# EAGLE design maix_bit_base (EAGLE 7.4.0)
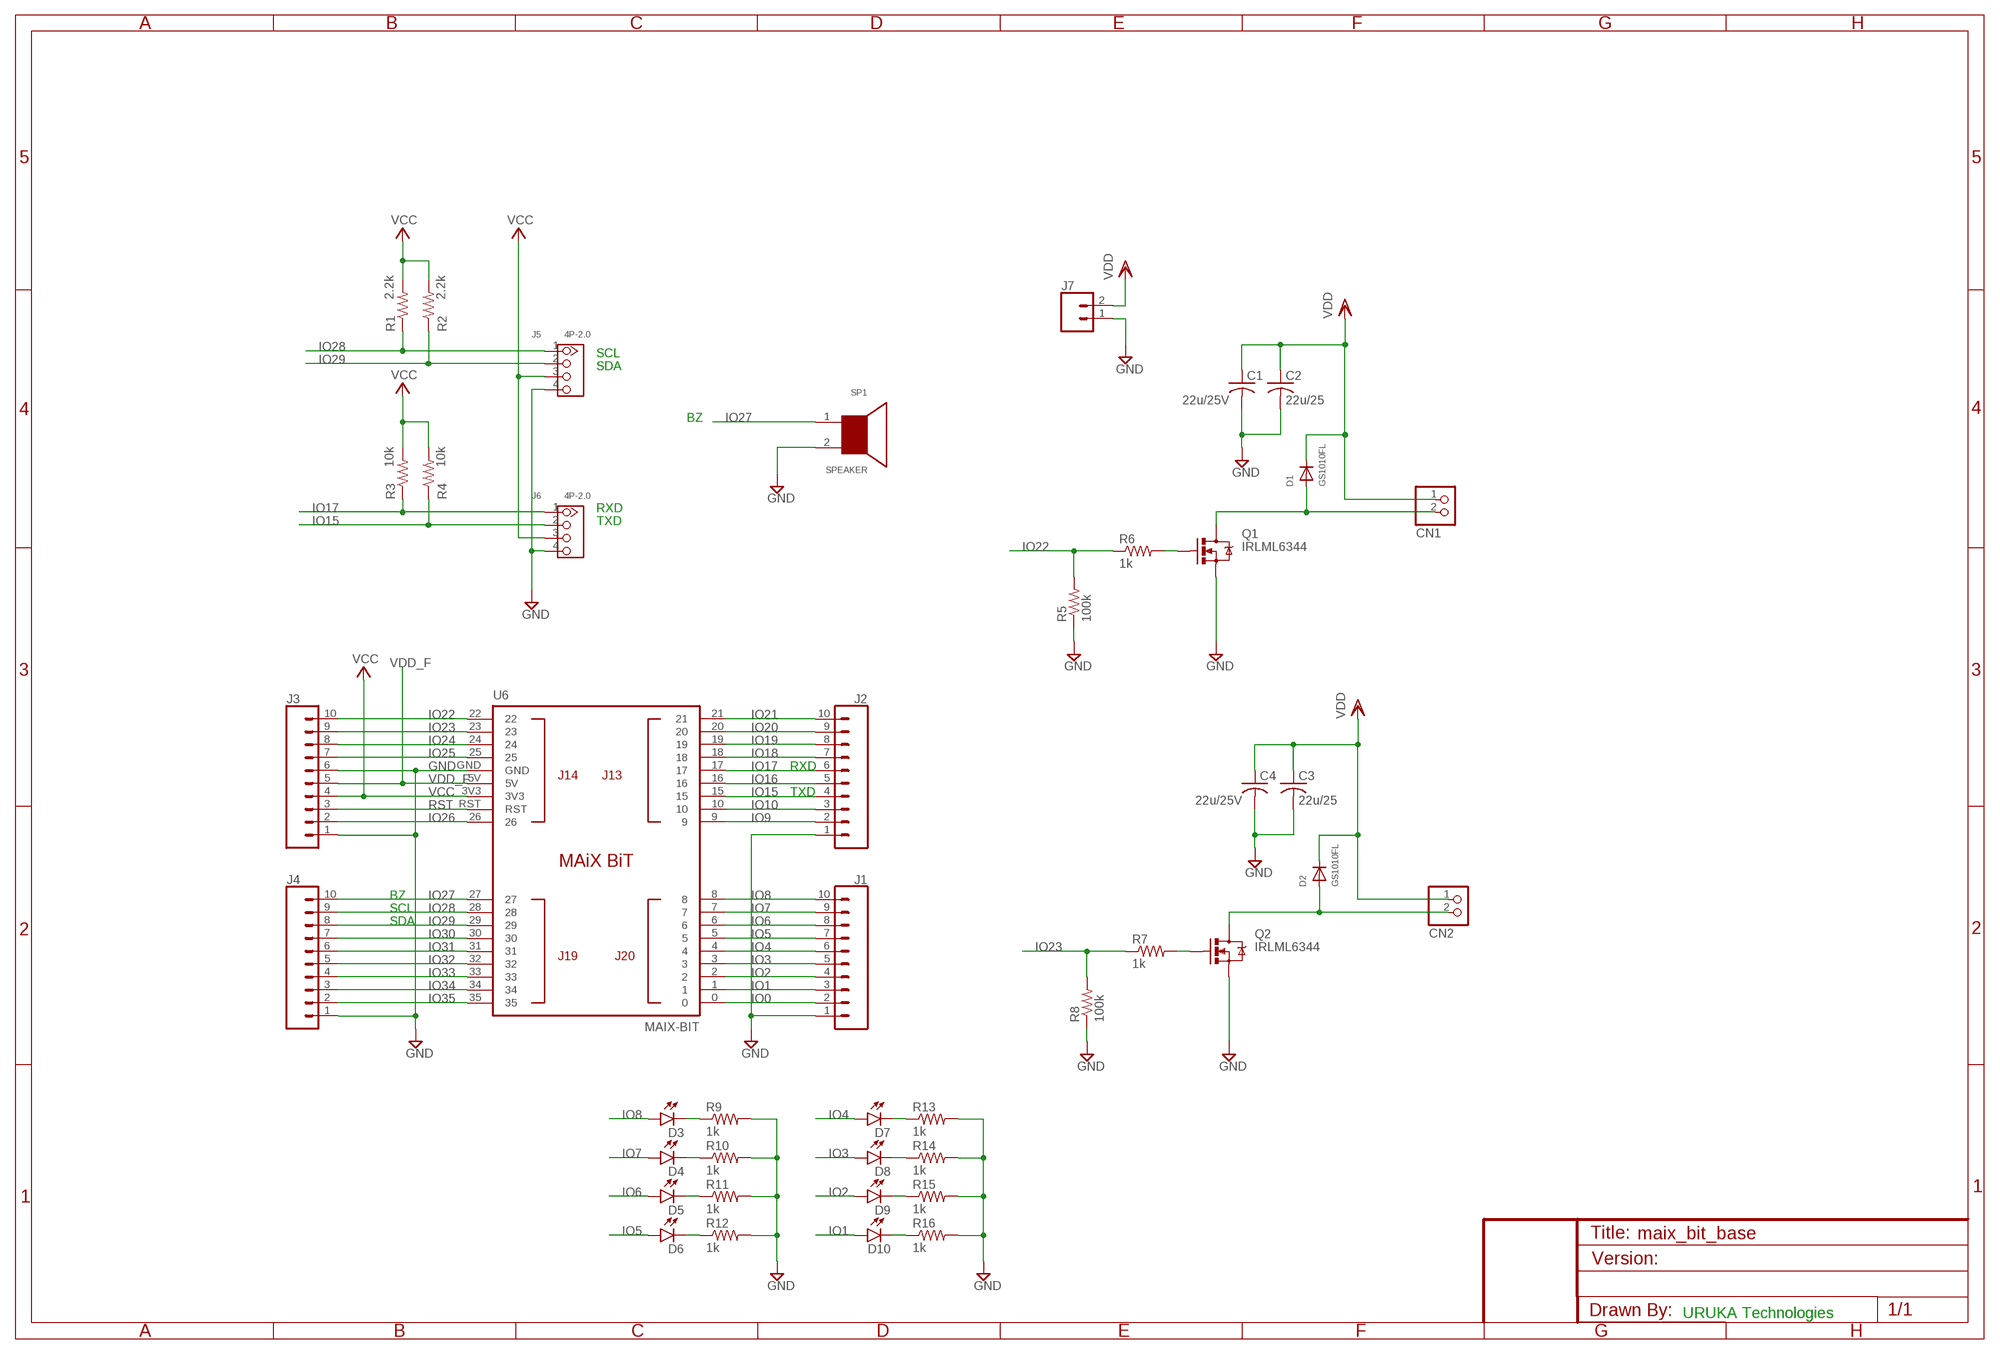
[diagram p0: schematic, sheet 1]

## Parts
C1  22u/25V  C-USC0805  [C0805]
C2  22u/25  C-USC0805  [C0805]
C3  22u/25  C-USC0805  [C0805]
C4  22u/25V  C-USC0805  [C0805]
CN1  JST_2PIN-SMT-RA  [JST-PH-2-SMT-RA]
CN2  JST_2PIN-SMT-RA  [JST-PH-2-SMT-RA]
D1  GS1010FL  [SOD-123FL]
D2  GS1010FL  [SOD-123FL]
D3  LED0603  [LED-0603]
D4  LED0603  [LED-0603]
D5  LED0603  [LED-0603]
D6  LED0603  [LED-0603]
D7  LED0603  [LED-0603]
D8  LED0603  [LED-0603]
D9  LED0603  [LED-0603]
D10  LED0603  [LED-0603]
J1  CONN_10"  [1X10]
J2  CONN_10"  [1X10]
J3  CONN_10"  [1X10]
J4  CONN_10"  [1X10]
J5  4P-2.0  GROVE-CONNECTOR-DIP(4P-2.0)  [HW4-2.0]
J6  4P-2.0  GROVE-CONNECTOR-DIP(4P-2.0)  [HW4-2.0]
J7  CONN_02  [1X02]
Q1  IRLML6344  MOSFET-NCHANNELBSS138  [SOT23-3]
Q2  IRLML6344  MOSFET-NCHANNELBSS138  [SOT23-3]
R1  2.2k  R-US_R0603  [R0603]
R2  2.2k  R-US_R0603  [R0603]
R3  10k  R-US_R0603  [R0603]
R4  10k  R-US_R0603  [R0603]
R5  100k  R-US_R0603  [R0603]
R6  1k  R-US_R0603  [R0603]
R7  1k  R-US_R0603  [R0603]
R8  100k  R-US_R0603  [R0603]
R9  1k  R-US_R0603  [R0603]
R10  1k  R-US_R0603  [R0603]
R11  1k  R-US_R0603  [R0603]
R12  1k  R-US_R0603  [R0603]
R13  1k  R-US_R0603  [R0603]
R14  1k  R-US_R0603  [R0603]
R15  1k  R-US_R0603  [R0603]
R16  1k  R-US_R0603  [R0603]
SP1  SPEAKER  [SPEAKER]
U6  MAIX-BIT  [MAIX-BIT]

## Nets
GND [power]: C1.2 C2.2 C3.2 C4.2 J1.1 J2.1 J3.1 J3.6 J4.1 J5.4 J6.4 J7.1 Q1.2(S) Q2.2(S) R5.1 R8.1 R9.2 R10.2 R11.2 R12.2 R13.2 R14.2 R15.2 R16.2 SP1.2 U6.GND
IO0: J1.2 U6.0
IO1: D10.A J1.3 U6.1
IO2: D9.A J1.4 U6.2
IO3: D8.A J1.5 U6.3
IO4: D7.A J1.6 U6.4
IO5: D6.A J1.7 U6.5
IO6: D5.A J1.8 U6.6
IO7: D4.A J1.9 U6.7
IO8: D3.A J1.10 U6.8
IO9: J2.2 U6.9
IO10: J2.3 U6.10
IO15: J2.4 J6.2 R4.1 U6.15
IO16: J2.5 U6.16
IO17: J2.6 J6.1 R3.1 U6.17
IO18: J2.7 U6.18
IO19: J2.8 U6.19
IO20: J2.9 U6.20
IO21: J2.10 U6.21
IO22: J3.10 R5.2 R6.1 U6.22
IO23: J3.9 R7.1 R8.2 U6.23
IO24: J3.8 U6.24
IO25: J3.7 U6.25
IO26: J3.2 U6.26
IO27: J4.10 SP1.1 U6.27
IO28: J4.9 J5.1 R1.1 U6.28
IO29: J4.8 J5.2 R2.1 U6.29
IO30: J4.7 U6.30
IO31: J4.6 U6.31
IO32: J4.5 U6.32
IO33: J4.4 U6.33
IO34: J4.3 U6.34
IO35: J4.2 U6.35
N$9: Q2.1(G) R7.2
N$10: Q1.1(G) R6.2
N$11 [moter]: CN1.2 D1.A Q1.3(D)
N$12 [moter]: CN2.2 D2.A Q2.3(D)
N$13: D4.C R10.1
N$14: D5.C R11.1
N$15: D6.C R12.1
N$16: D7.C R13.1
N$17: D8.C R14.1
N$18: D9.C R15.1
N$19: D10.C R16.1
N$20: D3.C R9.1
RST: J3.3 U6.RST
VCC [power]: J3.4 J5.3 J6.3 R1.2 R2.2 R3.2 R4.2 U6.3V3
VDD [moter]: C1.1 C2.1 C3.1 C4.1 CN1.1 CN2.1 D1.C D2.C J7.2
VDD_F [power]: J3.5 U6.5V

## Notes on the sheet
- SCL
- SDA
- BZ
- RXD
- TXD
- RXD
- TXD
- BZ
- SCL
- SDA
- URUKA Technologies

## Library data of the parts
C1-C4 = adafruit:C-US: CAPACITOR, American symbol
CN1 CN2 = solecon:JST_2PIN: JST 2-Pin Connectors of various flavors
D1 D2 = suna_power_device:GS1010FL
D3-D10 = SparkFun-LED:LED: LEDs
J1-J4 = SparkFun-Connectors:CONN_10: Multi connection point. Often used as Generic Header-pin footprint for 0.1 inch spaced/style header connections On any of the 0.1 inch spaced packages, you can populate with these: Break Away Headers - Straight (PRT-00116) Break Away Male Headers - Right Angle (PRT-00553) Female Headers (PRT-00115)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; PROD_ID: CONN-11563
J5 J6 = Seeed-OPL-Connector:GROVE-CONNECTOR-DIP(4P-2.0): 320110033
J7 = SparkFun-Connectors:CONN_02: Multi connection point. Often used as Generic Header-pin footprint for 0.1 inch spaced/style header connections
Q1 Q2 = SparkFun-DiscreteSemi:MOSFET-NCHANNEL: Common NMOSFET Parts MFG P/NStore IDProd ID FDD8780TRANS-09984 SI7820DNTRANS-11055 FDS6630AIC-08089 2N7002PWTRANS-11151 FQP30N06L COM-10213TRANS-10060 BSS123LT1GTRANS-08345 BSS138TRANS-00830 BS170 2N7000; PROD_ID: TRANS-00830; VALUE: 200mA/50V
R1-R16 = resistor:R-US_: RESISTOR, American symbol
SP1 = cq:SPEAKER
U6 = solecon:MAIX-BIT

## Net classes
1 power: width 0.762 mm, clearance 0.254 mm
2 Neopix: width 0.356 mm
3 moter: width 0.762 mm, clearance 0.254 mm

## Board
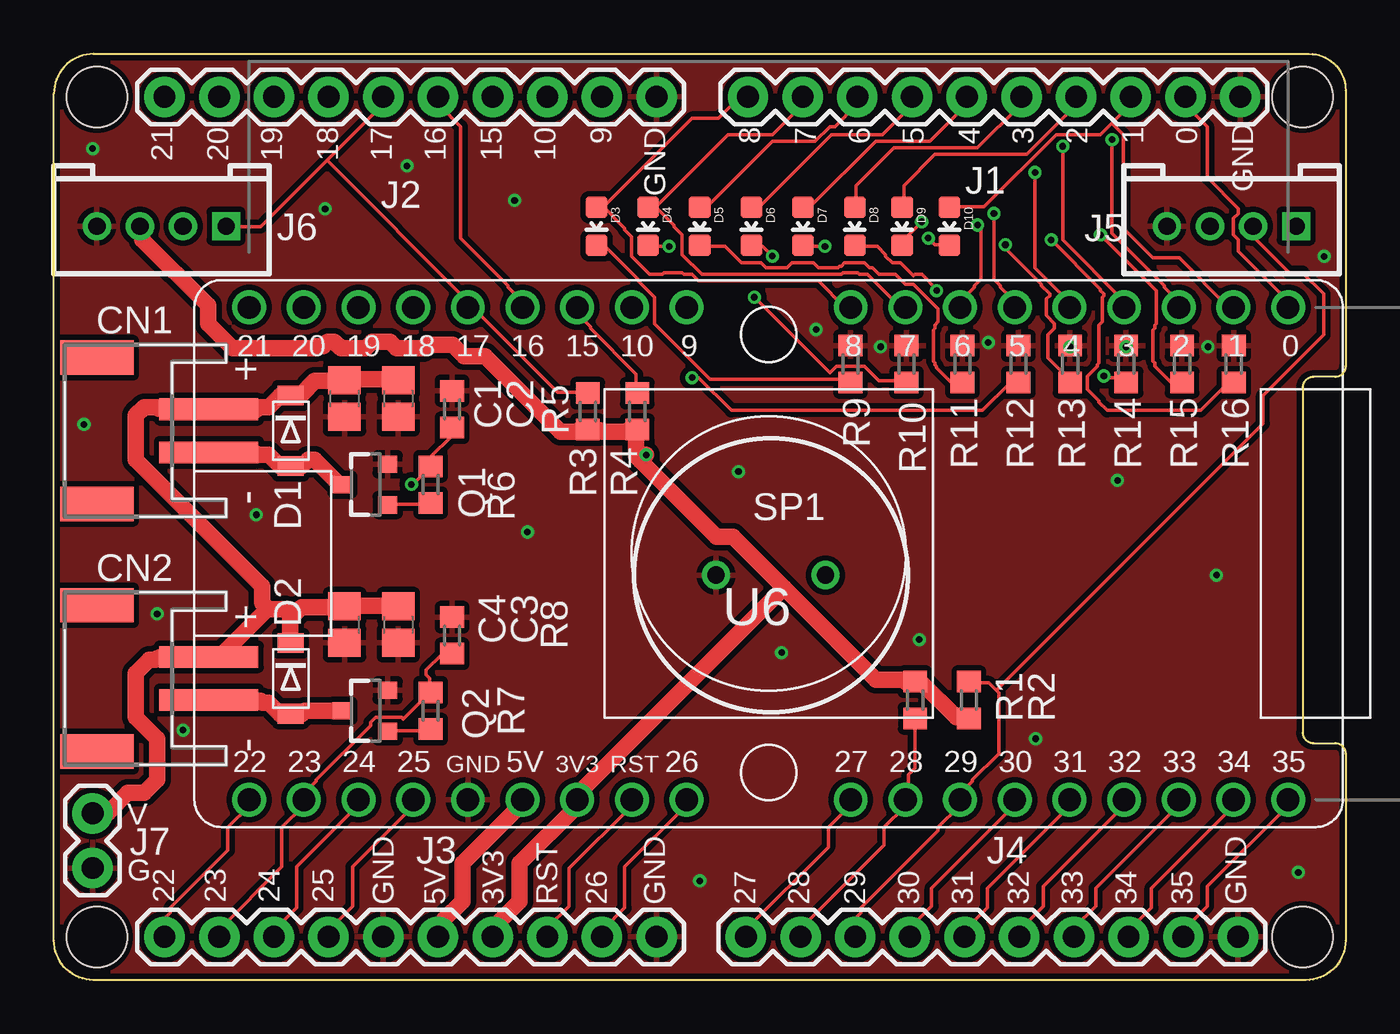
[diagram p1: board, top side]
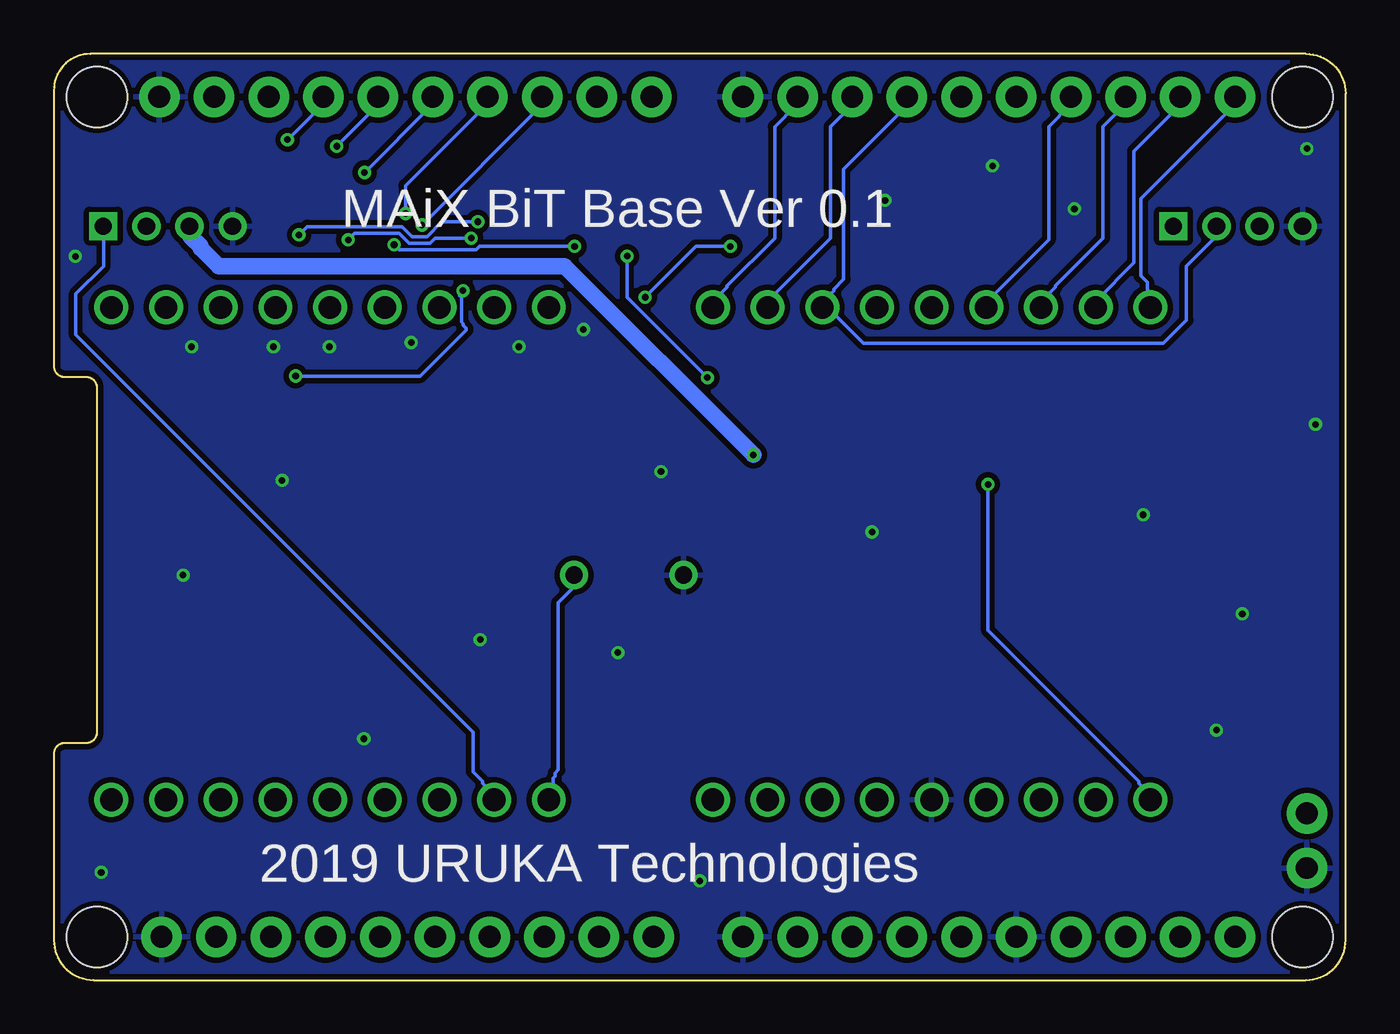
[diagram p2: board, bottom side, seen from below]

Size 60 x 43 mm. Coordinates in mm from the lower left corner, seen from the top.
Outline: 1.84,43 58.3,43 arc-90 60,41.3 60,28.5 arc-90 59.5,28 58.5,28 arc90 58,27.5 58,11.5 arc90 58.5,11 59.5,11 arc-90 60,10.5 60,1.84 arc-90 58.16,0 1.84,0 arc-90 0,1.84 0,41.16 arc-90 1.84,43
Copper layers (1*16): Top 0.035mm / dielectric 1.5mm / Bottom 0.035mm
Design rules "ssci_SeeedStudio_2layer_DRU_no_angle": minimum track width 6mil, minimum drill 12mil, track to track 6mil, track to pad 6mil, pad to pad 6mil, via to via 6mil, smd to smd 0mil, copper to edge 10mil, drill to drill 10mil, minimum pad ring 10mil, minimum via ring 6mil, stop-mask expansion 2mil, vias tented up to drill 25mil, thermal gap 10mil
Holes 2.8 mm at 2,41 2,2 58,2 58,41

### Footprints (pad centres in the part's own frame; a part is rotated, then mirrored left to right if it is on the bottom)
C0805 = smd 1.3 x 1.5: 1 -0.85,0; 2 0.85,0
JST-PH-2-SMT-RA = smd 1 x 4.6: 1 1,-3.7; 2 -1,-3.7 | smd 1.6 x 3.4: NC1 -3.4,1.5; NC2 3.4,1.5
SOD-123FL = smd 0.91 x 1.22: A 1.637,0; C -1.637,0
LED-0603 = smd 1 x 1: A 0,-0.877; C 0,0.877
1X10 = drill 1.016 pad 1.88: 1 0,0; 2 2.54,0; 3 5.08,0; 4 7.62,0; 5 10.16,0; 6 12.7,0; 7 15.24,0; 8 17.78,0; 9 20.32,0; 10 22.86,0
HW4-2.0 = drill 0.8 pad 1.27 square: 1 -3,0 | drill 0.8 pad 1.27: 2 -1,0; 3 1,0; 4 3,0
1X02 = drill 1.016 pad 1.88: 1 0,0; 2 2.54,0
SOT23-3 = smd 0.8 x 0.9: 1 -0.95,-1; 2 0.95,-1; 3 0,1.1
R0603 = smd 1 x 1.1: 1 -0.85,0; 2 0.85,0
SPEAKER = drill 0.8: 1 -2.54,0; 2 2.54,0
MAIX-BIT = drill 1.05: 0 24.13,11.43; 1 21.59,11.43; 2 19.05,11.43; 3 16.51,11.43; 3V3 -8.89,-11.43; 4 13.97,11.43; 5 11.43,11.43; 5V -11.43,-11.43; 6 8.89,11.43; 7 6.35,11.43; 8 3.81,11.43; 9 -3.81,11.43; 10 -6.35,11.43; 15 -8.89,11.43; 16 -11.43,11.43; 17 -13.97,11.43; 18 -16.51,11.43; 19 -19.05,11.43; 20 -21.59,11.43; 21 -24.13,11.43; 22 -24.13,-11.43; 23 -21.59,-11.43; 24 -19.05,-11.43; 25 -16.51,-11.43; 26 -3.81,-11.43; 27 3.81,-11.43; 28 6.35,-11.43; 29 8.89,-11.43; 30 11.43,-11.43; 31 13.97,-11.43; 32 16.51,-11.43; 33 19.05,-11.43; 34 21.59,-11.43; 35 24.13,-11.43; GND -13.97,-11.43; RST -6.35,-11.43

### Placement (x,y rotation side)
C1  13.5,27 270 top
C2  16,27 270 top
C3  16,16.5 270 top
C4  13.5,16.5 270 top
CN1  3.5,25.5 90 top
CN2  3.5,14 90 top
D1  11,25.5 270 top
D2  11,14 270 top
D3  25.2,35 180 top
D4  27.6,35 180 top
D5  30,35 180 top
D6  32.4,35 180 top
D7  34.8,35 180 top
D8  37.2,35 180 top
D9  39.4,35 180 top
D10  41.6,35 180 top
J1  55.1,41 180 top
J2  28,41 180 top
J3  28,2 180 top
J4  55,2 180 top
J5  54.7,35 180 top
J6  5,35 180 top
J7  1.8,5.2 90 top
Q1  14.5,23 90 top
Q2  14.5,12.5 90 top
R1  40,13 90 top
R2  42.5,13 270 top
R3  24.8,26.4 270 top
R4  27.1,26.4 270 top
R5  18.5,26.5 270 top
R6  17.5,23 270 top
R7  17.5,12.5 270 top
R8  18.5,16 270 top
R9  37,28.6 90 top
R10  39.6,28.6 90 top
R11  42.2,28.6 90 top
R12  44.8,28.6 90 top
R13  47.2,28.6 90 top
R14  49.8,28.6 90 top
R15  52.4,28.6 90 top
R16  54.8,28.6 90 top
SP1  33.3,18.8 180 top
U6  33.2,19.8 0 top

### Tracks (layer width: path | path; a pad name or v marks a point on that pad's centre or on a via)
GND  (via drill 0.3)
  other vias: 1.8,38.6 16.4,37.8 21.4,36.2 12.6,35.8 1.4,25.8 9.4,21.6 22,20.8 31.8,23.6 49.4,23.2 54,18.8 40.2,15.8 33.8,15.2 30,4.6 57.8,5 6,11.6 4.8,17 59,33.6 45.6,11.2 43.4,29.6 53.6,29.4 38.4,29.4 35.4,30.2 49.8,29.4 47.2,29.4
  pour Top: 0,0 60,0 60,43 0,43
  pour Bottom: 0,0 60,0 60,43 0,43
IO0
  Top 0.152: U6.0 57.3,31.24 57.3,31.55 55.02,33.83 55.02,34.37 54.79,34.59 54.79,35.36 55.02,35.59 55.02,35.81 53.57,37.26 53.57,39.62 52.58,40.62 52.58,41 J1.2
IO1
  Top 0.152: 49.15,39.78 49.99,40.62 49.99,41 J1.3 | 49.15,39.78 48.62,39.24 46.56,39.24 43.2,35.89 D10.A | 49.15,39.78 49.68,39.24 49.68,34.9 51.05,33.53 52.27,33.53 54.56,31.24 54.79,31.24 U6.1
IO2  (via drill 0.3)
  Top 0.152: D9.A 39.47,35.89 39.47,36.88 40.92,38.33 45.19,38.33 47.47,40.62 J1.4 | v49.15,39.01 49.15,34.67 51.59,32.23 51.59,32.16 52.2,31.55 52.2,31.24 U6.2
  Bottom 0.152: v49.15,39.01 47.55,40.62 47.55,41 J1.4
IO3  (via drill 0.3)
  Top 0.152: D8.A 37.26,35.89 37.26,36.88 39.01,38.63 42.9,38.63 44.88,40.62 44.88,41 J1.5 | v46.86,38.71 46.86,34.37 49.68,31.55 49.68,31.24 U6.3
  Bottom 0.152: v46.86,38.71 44.96,40.62 44.96,41 J1.5
IO4  (via drill 0.3)
  Top 0.152: D7.A 34.82,35.89 35.13,35.89 38.18,38.94 40.69,38.94 42.37,40.62 42.37,41 J1.6 | v45.57,37.49 45.57,33.07 47.17,31.47 47.17,31.24 U6.4
  Bottom 0.152: v45.57,37.49 42.44,40.62 42.44,41 J1.6
IO5  (via drill 0.3)
  Top 0.152: D6.A 32.46,35.89 32.77,35.89 36.12,39.24 38.48,39.24 39.85,40.62 J1.7 | v43.66,35.59 43.66,32.54 43.97,32.23 43.97,32.16 44.58,31.55 44.58,31.24 U6.5
  Bottom 0.152: v43.66,35.59 43.66,36.88 39.93,40.62 39.93,41 J1.7
IO6  (via drill 0.3)
  Top 0.152: D5.A 30.02,35.89 30.33,35.89 33.38,38.94 35.36,38.94 36.04,39.62 36.27,39.62 37.26,40.62 37.26,41 J1.8 | v42.9,35.05 43.05,34.9 43.05,32.54 42.75,32.23 42.75,32.16 42.14,31.55 42.14,31.24 U6.6
  Bottom 0.152: v42.9,35.05 37.34,40.62 37.34,41 J1.8
IO7
  Top 0.152: 27.89,35.89 27.96,35.89 31.32,39.24 33.38,39.24 34.75,40.62 34.75,41 J1.9 | 27.89,35.89 27.66,35.89 D4.A 27.89,35.89 | 27.89,35.89 27.96,35.81 28.04,35.81 28.8,35.05 28.8,34.98 29.18,34.59 29.18,33.68 30.1,32.77 36.58,32.77 36.65,32.84 37.34,32.84 37.41,32.77 37.8,32.77 39.32,31.24 39.55,31.24 U6.7
IO8
  Top 0.152: 25.53,35.89 25.22,35.89 D3.A 25.53,35.89 | 25.53,35.89 29.64,40.01 30.86,40.01 31.85,41 J1.10 | 25.53,35.89 26.52,34.9 26.52,34.82 26.82,34.52 26.82,33.6 27.66,32.77 28.27,32.77 28.35,32.84 29.18,32.84 29.26,32.77 29.64,32.77 29.95,32.46 35.51,32.46 36.73,31.24 36.96,31.24 U6.8
IO9
  Bottom 0.152: U6.9 29.34,31.24 29.34,31.55 28.73,32.16 28.73,32.23 26.52,34.44 26.52,39.62 25.53,40.62 25.53,41 J2.2
IO10
  Bottom 0.152: U6.10 26.82,31.24 26.82,31.55 23.93,34.44 23.93,39.62 22.94,40.62 22.94,41 J2.3
IO15
  Top 0.152: R4.1 27.05,27.28 27.05,28.12 24.92,30.25 24.92,30.33 24.38,30.86 24.38,31.17 U6.15
  Bottom 0.152: J6.2 6.02,34.98 6.02,34.52 7.39,33.15 7.39,30.63 8.46,29.57 22.4,29.57 24,31.17 24.31,31.17 U6.15 23.93,31.17 23.93,31.85 23.77,32 23.77,32.08 23.32,32.54 23.32,37.64 20.42,40.54 20.42,41 J2.4
IO16
  Top 0.152: U6.16 21.72,31.24 21.72,31.55 21.11,32.16 21.11,32.23 18.9,34.44 18.9,39.62 17.91,40.62 17.91,41 J2.5
IO17
  Top 0.152: R3.1 24.77,27.28 23.39,27.28 19.51,31.17 19.28,31.17 U6.17 19.2,31.24 19.2,31.55 12.69,38.06 | 12.69,38.06 15.24,40.62 15.24,41 J2.6 | 12.69,38.06 9.6,34.98 8,34.98 J6.1
IO18
  Bottom 0.152: U6.18 16.69,31.24 16.69,31.47 13.79,34.37 13.79,39.62 12.8,40.62 12.8,41 J2.7
IO19
  Bottom 0.152: U6.19 14.1,31.24 14.1,31.55 13.49,32.16 13.49,32.23 11.28,34.44 11.28,39.62 10.29,40.62 10.29,41 J2.8
IO20
  Bottom 0.152: U6.20 11.58,31.24 11.58,31.55 9.83,33.3 9.83,38.48 7.7,40.62 7.7,41 J2.9
IO21
  Bottom 0.152: U6.21 9.14,31.24 9.14,32 9.22,32.08 9.22,32.38 9.53,32.69 9.53,36.27 5.18,40.62 5.18,41 J2.10
IO22  (via drill 0.3)
  Top 0.152: R5.2 18.44,25.6 18.44,25.22 17.53,24.31 17.53,23.85 R6.1 17.45,23.77 16.69,23.01 v16.61,23.01 | J3.10 5.18,2.06 5.18,2.9 5.41,3.12 5.41,3.35 8.08,6.02 8.08,7.09 9.07,8.08 9.07,8.31 U6.22
  Bottom 0.152: v16.61,23.01 16.61,16.23 9.6,9.22 9.6,9.14 9.14,8.69 9.14,8.38 U6.22
IO23
  Top 0.152: R8.2 18.44,15.09 17.98,15.09 17.3,14.4 17.3,14.17 17.45,14.02 17.45,13.41 R7.1 17.45,13.34 16.23,12.12 16.15,12.19 14.94,12.19 14.71,11.96 14.71,11.81 12.19,9.3 12.19,9.22 11.66,8.69 11.66,8.38 U6.23 11.58,8.31 11.58,8.08 10.59,7.09 10.59,5.26 7.7,2.36 7.7,2.06 J3.9
IO24
  Top 0.152: U6.24 14.1,8.31 14.1,8.08 11.28,5.26 11.28,3.35 10.29,2.36 10.29,2.06 J3.8
IO25
  Top 0.152: U6.25 16.69,8.31 16.69,8.08 13.87,5.26 13.87,3.43 12.8,2.36 12.8,2.06 J3.7
IO26
  Top 0.152: U6.26 29.34,8.31 29.34,8.08 26.52,5.26 26.52,3.35 25.53,2.36 25.53,2.06 J3.2
IO27
  Top 0.152: J4.10 32.16,2.06 32.16,2.36 35.97,6.17 35.97,7.09 36.96,8.08 36.96,8.31 U6.27
  Bottom 0.152: SP1.1 35.89,18.75 35.89,18.21 36.58,17.53 36.58,9.75 36.73,9.6 36.73,9.45 36.8,9.37 36.8,9.14 36.96,8.99 36.96,8.38 U6.27
IO28
  Top 0.152: R1.1 40.01,12.12 40.01,9.83 39.7,9.53 39.7,8.46 39.62,8.38 U6.28 39.55,8.31 39.55,8.08 38.56,7.09 38.56,6.25 34.75,2.44 34.75,2.06 J4.9
  Bottom 0.152: J5.1 57.68,34.98 57.68,33.15 58.98,31.85 58.98,29.95 40.54,11.51 40.54,9.68 40.08,9.22 40.08,9.14 39.62,8.69 39.62,8.38 U6.28
IO29
  Top 0.152: 43.78,13.45 43.89,13.34 43.89,10.52 42.67,9.3 42.67,9.22 42.14,8.69 42.14,8.38 U6.29 42.06,8.31 42.06,8.08 41.07,7.09 41.07,6.93 37.49,3.35 37.49,3.12 37.26,2.9 37.26,2.06 J4.8 | 43.78,13.45 43.43,13.79 42.52,13.79 R2.1 | 43.78,13.45 56.16,25.83 56.16,27.13 58.98,29.95 58.98,31.85 57.99,32.84 57.38,32.84 55.7,34.52 55.7,34.98 J5.2
IO30
  Top 0.152: U6.30 44.58,8.31 44.58,8.08 40.77,4.27 40.77,3.43 39.78,2.44 39.78,2.06 J4.7
IO31
  Top 0.152: U6.31 47.17,8.31 47.17,8.08 43.36,4.27 43.36,3.35 42.37,2.36 42.37,2.06 J4.6
IO32
  Top 0.152: U6.32 49.68,8.31 49.68,8.08 45.95,4.34 45.95,3.43 44.88,2.36 44.88,2.06 J4.5
IO33
  Top 0.152: U6.33 52.2,8.31 52.2,8.08 48.39,4.27 48.39,3.43 47.4,2.44 47.4,2.06 J4.4
IO34
  Top 0.152: U6.34 54.79,8.31 54.79,8.08 50.98,4.27 50.98,3.35 49.99,2.36 49.99,2.06 J4.3
IO35
  Top 0.152: U6.35 57.3,8.31 57.3,8.08 53.57,4.34 53.57,3.43 52.5,2.36 52.5,2.06 J4.2
N$9
  Top 0.152: Q2.1 15.54,11.58 17.45,11.58 R7.2
N$10
  Top 0.152: Q1.1 15.54,22.1 17.45,22.1 R6.2
N$11
  Top 0.762: Q1.3 13.34,23.01 13.26,23.01 12.12,24.16 11.81,24.16 11.51,23.85 11.05,23.85 D1.A 10.67,23.85 10.52,23.85 9.98,24.38 9.45,24.38 9.37,24.46 7.24,24.46 CN1.2
N$12
  Top 0.762: Q2.3 13.34,12.5 11.66,12.5 11.51,12.34 11.05,12.34 D2.A 10.59,12.34 10.52,12.34 9.98,12.88 9.68,12.88 9.6,12.95 7.24,12.95 CN2.2
N$13  (via drill 0.3)
  Top 0.152: v28.57,34.06 27.66,34.06 D4.C | v32.54,31.7 36.04,28.19 36.35,28.5 37.64,28.5 38.33,27.81 39.55,27.81 R10.1
  Bottom 0.152: v28.57,34.06 30.18,34.06 v32.54,31.7
N$14
  Top 0.152: D5.C 30.02,34.06 31.17,34.06 31.93,33.3 32.84,33.3 33.07,33.07 34.06,33.07 34.29,33.3 35.28,33.3 35.51,33.07 36.42,33.07 36.5,33.15 36.58,33.15 36.73,33.3 37.64,33.3 37.87,33.07 38.02,33.07 38.33,32.77 39.09,32.77 39.55,32.31 39.93,32.31 41.07,31.17 41.07,30.56 40.92,30.4 40.92,30.25 40.84,30.18 40.84,28.73 40.92,28.65 40.92,28.57 41,28.5 41,28.42 41.68,27.74 42.14,27.74 R11.1
N$15  (via drill 0.3)
  Top 0.152: v33.38,33.6 32.92,34.06 32.46,34.06 D6.C | v29.64,27.96 29.95,27.96 31.47,26.44 43.13,26.44 44.42,27.74 44.73,27.74 R12.1
  Bottom 0.152: v33.38,33.6 33.38,31.7 v29.64,27.96
N$16  (via drill 0.3)
  Top 0.152: v35.81,34.06 34.82,34.06 D7.C | v44.2,34.14 44.2,33.98 45.87,32.31 45.87,32.23 46.25,31.85 46.25,31.77 46.1,31.62 46.1,30.86 46.48,30.48 46.48,30.25 46.18,29.95 46.18,28.88 47.24,27.81 R13.1
  Bottom 0.152: v35.81,34.06 40.23,34.06 40.39,33.91 43.97,33.91 v44.2,34.14
N$17  (via drill 0.3)
  Top 0.152: v41,32 41,32.08 40.31,32.77 40.01,32.77 39.93,32.69 39.32,33.3 38.94,33.3 38.63,33.6 38.63,33.68 38.25,34.06 37.26,34.06 D8.C | v48.77,28.04 48.84,27.96 49.61,27.96 49.76,27.81 R14.1
  Bottom 0.152: v41,32 41.15,31.85 41.15,31.77 41.07,31.7 41.07,30.56 41,30.48 41,30.4 40.84,30.25 40.84,30.18 42.98,28.04 v48.77,28.04
N$18  (via drill 0.3)
  Top 0.152: v40.31,35.2 39.47,34.37 39.47,34.14 D9.C | v48.62,34.59 51.21,32 51.21,30.48 51.13,30.4 51.13,30.25 51.05,30.18 51.05,28.73 51.13,28.65 51.13,28.5 51.89,27.74 52.35,27.74 R15.1
  Bottom 0.152: v40.31,35.2 41.99,35.2 42.67,34.52 43.36,34.52 43.81,34.98 48.23,34.98 v48.62,34.59
N$19  (via drill 0.3)
  Top 0.152: v40.62,34.44 40.92,34.14 41.53,34.14 D10.C | v46.33,34.37 48.62,32.08 48.62,32 48.77,31.85 48.77,31.77 48.69,31.7 48.69,30.56 48.54,30.4 48.54,28.65 48.46,28.57 48.46,28.5 48.01,28.04 48.01,27.43 48.54,26.9 48.54,26.82 48.92,26.44 53.26,26.44 54.56,27.74 54.79,27.74 R16.1
  Bottom 0.152: v40.62,34.44 42.29,34.44 42.52,34.21 43.51,34.21 43.97,34.67 46.02,34.67 v46.33,34.37
N$20
  Top 0.152: D3.C 25.22,34.06 25.6,34.06 27.13,32.54 27.13,32.46 27.89,31.7 27.89,30.48 30.48,27.89 36.88,27.89 36.96,27.81 R9.1
RST
  Top 0.152: U6.RST 26.82,8.31 26.82,8.08 23.93,5.18 23.93,3.43 22.94,2.44 22.94,2.06 J3.3
VCC  (via drill 0.3)
  Top 0.762: J3.4 20.42,2.06 20.42,2.44 21.64,3.66 21.64,5.41 24.31,8.08 24.31,8.31 U6.3V3 24.46,8.69 24.46,8.76 33.91,18.21 | R2.2 42.44,12.19 41.91,12.19 40.23,13.87 40.01,13.87 R1.2 39.62,13.79 39.47,13.95 38.18,13.95 33.91,18.21 | 27.24,24.12 30.79,20.57 31.55,20.57 33.91,18.21 | 27.24,24.12 27.05,24.31 27.05,25.15 R4.2 27.05,25.53 26.67,25.53 26.59,25.45 25.45,25.45 25.38,25.53 24.84,25.53 R3.2 24.46,25.6 24.31,25.45 23.55,25.45 20.04,28.96 19.05,28.96 18.52,29.49 17.3,29.49 17.14,29.34 15.93,29.34 15.62,29.64 14.78,29.64 14.48,29.34 13.34,29.34 13.03,29.64 12.72,29.64 12.5,29.41 12.19,29.41 12.12,29.34 8.31,29.34 7.16,30.48 7.16,31.32 4.12,34.37 4.12,34.52 4.04,34.59 4.04,34.98 J6.3 | v27.51,24.38 27.24,24.12
  Bottom 0.762: v27.51,24.38 36.27,33.15 52.35,33.15 53.19,33.98 53.19,34.06 53.65,34.52 53.65,34.98 J5.3
VDD
  Top 0.762: C2.1 15.93,27.89 13.95,27.89 13.79,28.04 C1.1 13.49,27.81 12.12,27.81 11.51,27.2 11.05,27.2 D1.C 10.67,27.13 10.52,27.13 9.98,26.59 9.53,26.59 9.37,26.44 7.24,26.44 CN1.1 6.86,26.52 4.88,26.52 4.8,26.59 4.19,26.59 3.81,26.21 3.81,24.16 9.68,18.29 9.68,17.53 9.91,17.22 | 11.09,16.88 11.51,17.3 13.49,17.3 C4.1 13.87,17.37 15.93,17.37 C3.1 | 11.09,16.88 10.97,16.76 10.97,15.7 D2.C | 9.91,17.22 10.74,17.22 11.09,16.88 | 9.91,17.22 7.7,15.01 7.24,15.01 CN2.1 6.86,15.01 4.95,15.01 4.88,14.94 4.8,14.94 4.72,14.86 4.42,14.86 3.81,14.25 3.81,12.19 4.8,11.2 4.8,9.3 4.19,8.69 3.43,8.69 2.52,7.77 1.83,7.77 J7.2
VDD_F
  Top 0.762: U6.5V 21.72,8.31 21.72,8.15 18.97,5.41 18.97,3.66 18.14,2.82 18.14,2.74 17.91,2.52 17.91,2.06 J3.5

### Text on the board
tPlace: 21 | 20 | 19 | 18 | 17 | 16 | 15 | 10 | 9 | GND | 8 | 7 | 6 | 5 | 4 | 3 | 2 | 1 | 0 | GND | V | G | 22 | 23 | 24 | 25 | GND | 5V | 3V3 | RST | 26 | GND | 27 | 28 | 29 | 30 | 31 | 32 | 33 | 34 | 35 | GND
bPlace: MAiX BiT Base Ver 0.1 | 2019 URUKA Technologies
